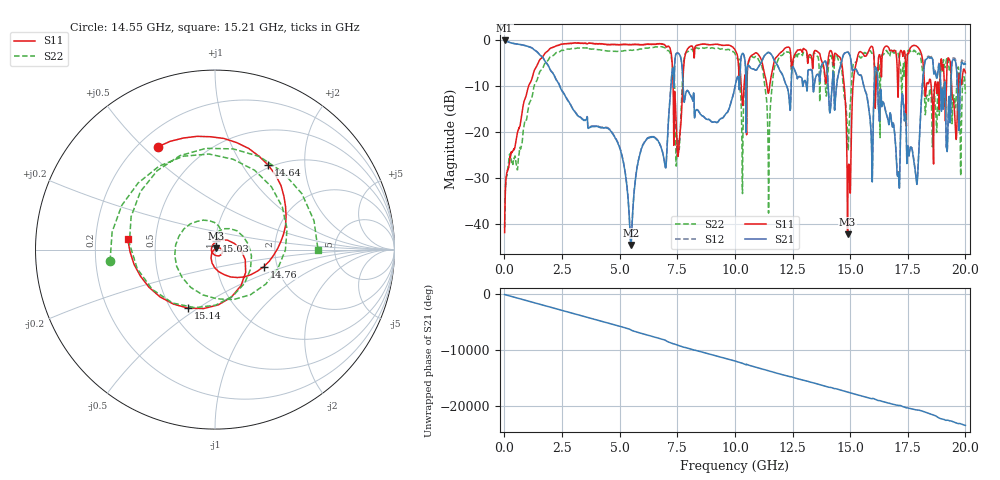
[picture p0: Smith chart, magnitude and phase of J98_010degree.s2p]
!Keysight Technologies,N5222A,MY51421036,A.10.65.16
!Date: Friday, March 31, 2023 14:39:21
!Correction: S11(Full 2 Port(1,2))
!S21(Full 2 Port(1,2))
!S12(Full 2 Port(1,2))
!S22(Full 2 Port(1,2))
!S2P File: Measurements: S11, S21, S12, S22:
# Hz S  dB  R 50
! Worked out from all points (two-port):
!   2000 points, 10 MHz to 20 GHz, reference 50 ohm
!   highest |S21| = -0.03 dB at 10 MHz (marker M1); lowest = -44.6 dB at 5.49 GHz (marker M2)
!   |S21| within 3 dB of the highest: start of sweep to 1.51 GHz; 14.73 GHz to 14.97 GHz (239.3 MHz wide, 1.61 % of centre)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
!   lowest |S11| = -42.3 dB at 14.89 GHz (marker M3), VSWR 1.02, Z = 50.4 + j0.66 ohm
!   |S11| at or under -10 dB: start of sweep to 1.047 GHz; 7.32 GHz to 7.734 GHz (414.7 MHz wide, 5.51 % of centre); 14.75 GHz to 15.12 GHz (377.2 MHz wide, 2.53 % of centre)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
!   |S22| runs from -40.9 to -1.4 dB; largest |S21 - S12| = 0.043
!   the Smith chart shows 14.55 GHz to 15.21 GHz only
!   S11 on the Smith chart (normalised r, x): 14.55 GHz: 0.28, +0.55; 14.64 GHz: 0.96, +1.31; 14.76 GHz: 1.70, -0.35; 15.03 GHz: 1.01, +0.09; 15.14 GHz: 0.61, -0.46; 15.21 GHz: 0.34, +0.05
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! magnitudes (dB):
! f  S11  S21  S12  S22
! 10 MHz  -41.9  0.0  -0.1  -40.9
! 1.37 GHz  -5.9  -2.3  -2.3  -9.1
! 3.35 GHz  -0.6  -17.0  -16.9  -1.7
! 5.49 GHz  -0.9  -44.6  -44.9  -2.1
! 6.68 GHz  -0.8  -22.0  -21.9  -1.5
! 7.53 GHz  -25.3  -2.8  -2.7  -21.3
! 7.9 GHz  -2.4  -11.1  -11.1  -2.6
! 10.01 GHz  -2.1  -10.0  -10.0  -3.0
! 11.47 GHz  -11.3  -2.7  -2.6  -33.0
! 13.34 GHz  -4.1  -6.5  -6.5  -4.0
! 14.55 GHz  -3.7  -6.2  -6.1  -4.6
! 14.64 GHz  -5.1  -4.4  -4.3  -6.5
! 14.76 GHz  -10.8  -2.8  -2.7  -12.7
! 14.89 GHz  -42.3  -2.6  -2.5  -21.5
! 15.03 GHz  -26.5  -4.2  -4.2  -12.0
! 15.14 GHz  -8.9  -6.5  -6.4  -5.1
! 15.21 GHz  -6.2  -6.3  -6.2  -4.8
! 16.67 GHz  -1.6  -18.1  -18.0  -3.0
! 17.86 GHz  -1.2  -30.2  -30.0  -2.7
! 18.31 GHz  -9.8  -4.1  -3.8  -12.3
! 19.25 GHz  -3.9  -16.8  -16.6  -4.4
! 20 GHz  -7.1  -5.1  -4.7  -11.6
